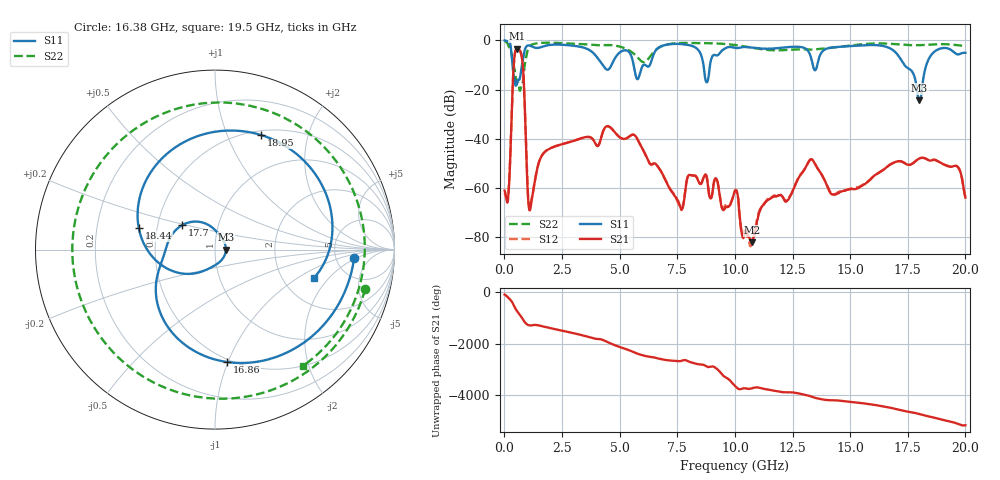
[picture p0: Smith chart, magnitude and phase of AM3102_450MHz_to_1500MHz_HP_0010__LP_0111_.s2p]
!Agilent Technologies,E8364B,MY43040894,A.07.50.67
!Agilent E8364B: A.07.50.67
!Date: Thursday, January 11, 2018 05:25:27
!Correction: S11(Full 2 Port(1,2))
!S21(Full 2 Port(1,2))
!S12(Full 2 Port(1,2))
!S22(Full 2 Port(1,2))
!S2P File: Measurements: S11, S21, S12, S22:
# Hz S  dB  R 50
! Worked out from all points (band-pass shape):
!   1601 points, 10 MHz to 20 GHz, reference 50 ohm
!   highest |S21| = -3.44 dB at 559.7 MHz (marker M1); lowest = -82.0 dB at 10.74 GHz (marker M2)
!   |S21| within 3 dB of the highest: 440.6 MHz to 750.4 MHz (309.8 MHz wide, 52 % of centre)
!   lowest |S11| = -24.4 dB at 18 GHz (marker M3), VSWR 1.13, Z = 56.4 + j0.0521 ohm
!   |S11| at or under -10 dB: 351.3 MHz to 763.3 MHz (412 MHz wide, 73.9 % of centre); 5.607 GHz to 6.038 GHz (431.2 MHz wide, 7.41 % of centre); 17.35 GHz to 18.31 GHz (952.6 MHz wide, 5.34 % of centre)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
!   |S22| runs from -20.5 to -0.4 dB; largest |S21 - S12| = 0.0027
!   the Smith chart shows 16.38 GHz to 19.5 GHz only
!   S11 on the Smith chart (normalised r, x): 16.38 GHz: 7.48, -1.83; 16.86 GHz: 0.48, -0.99; 17.7 GHz: 0.67, +0.19; 18.44 GHz: 0.39, +0.12; 18.95 GHz: 0.55, +1.33; 19.5 GHz: 2.99, -1.39
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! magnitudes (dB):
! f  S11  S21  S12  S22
! 10 MHz  -0.1  -61.0  -62.0  -0.4
! 172.4 MHz  -0.6  -62.9  -62.3  -2.1
! 559.7 MHz  -17.2  -3.4  -3.4  -17.1
! 784.6 MHz  -8.9  -8.7  -8.7  -17.2
! 1.109 GHz  -2.2  -69.0  -68.4  -2.3
! 1.697 GHz  -2.4  -45.9  -45.9  -1.0
! 3.346 GHz  -2.7  -39.7  -39.7  -1.5
! 6.682 GHz  -3.0  -51.6  -51.6  -3.1
! 7.644 GHz  -1.5  -68.0  -68.0  -1.1
! 8.781 GHz  -17.1  -55.7  -55.5  -1.2
! 10.01 GHz  -3.1  -61.2  -60.9  -1.9
! 10.74 GHz  -3.0  -82.0  -81.9  -3.0
! 13.34 GHz  -8.4  -48.3  -48.4  -3.8
! 16.38 GHz  -2.2  -53.0  -53.0  -1.3
! 16.68 GHz  -3.0  -50.8  -50.8  -1.4
! 16.86 GHz  -4.0  -49.8  -49.8  -1.5
! 17.7 GHz  -12.9  -50.1  -50.1  -2.0
! 18 GHz  -24.4  -48.0  -48.0  -2.0
! 18.44 GHz  -7.1  -48.8  -48.7  -1.8
! 18.95 GHz  -3.2  -49.9  -49.8  -1.6
! 19.5 GHz  -4.8  -51.1  -51.0  -1.8
! 20 GHz  -5.1  -63.9  -63.7  -2.4
